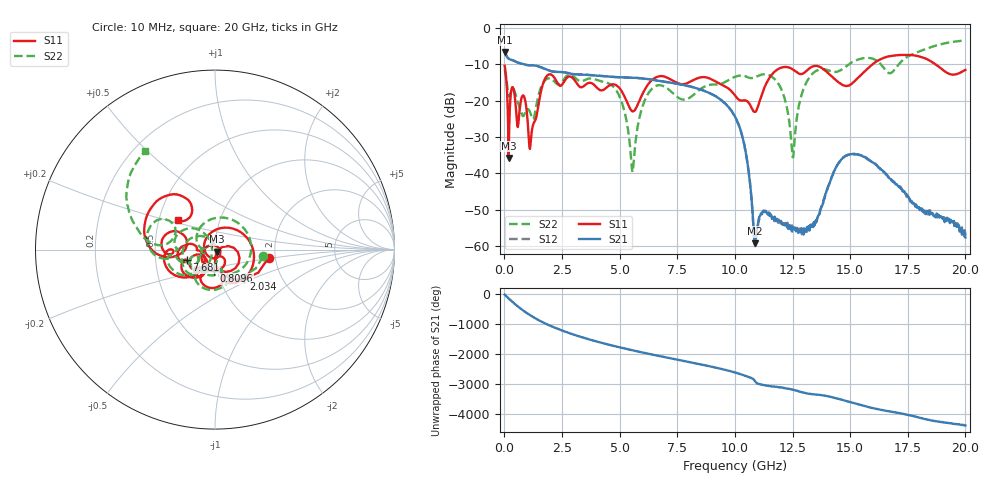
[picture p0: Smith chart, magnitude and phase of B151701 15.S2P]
!  2-Port S-parameters saved by WinCal
! VAR MeasName=S-Parameters (CALIBRATED_DATA) read from VNA (N5244A)
! VAR MeasDate=2015-12-24 19:09:51
! VAR NAME=B151701 15
! VAR FILENAME=B151701 15.S2P
! VAR DATE=2015-12-24 19:09:51
! VAR PHYS_PORTS=1,3
# Hz S DB R 50
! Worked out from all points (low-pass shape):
!   801 points, 10 MHz to 20 GHz, reference 50 ohm
!   highest |S21| = -6.63 dB at 10 MHz (marker M1); lowest = -59.3 dB at 10.85 GHz (marker M2)
!   |S21| within 3 dB of the highest: start of sweep to 635.4 MHz
!   lowest |S11| = -35.7 dB at 184.9 MHz (marker M3), VSWR 1.03, Z = 51.1 - j1.19 ohm
!   |S11| at or under -10 dB: start of sweep to 15.98 GHz; 18.7 GHz to end of sweep
!   |S22| runs from -39.6 to -3.5 dB; largest |S21 - S12| = 0.0013
!   S11 on the Smith chart (normalised r, x): 10 MHz: 1.84, -0.18; 809.6 MHz: 0.96, -0.23; 2.034 GHz: 1.30, -0.44; 7.681 GHz: 0.72, -0.09; 20 GHz: 0.63, +0.22
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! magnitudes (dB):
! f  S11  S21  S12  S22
! 10 MHz  -10.4  -6.6  -6.7  -11.3
! 184.9 MHz  -35.7  -8.4  -8.4  -18.4
! 809.6 MHz  -18.6  -9.9  -9.9  -24.3
! 1.134 GHz  -31.9  -10.3  -10.3  -23.5
! 2.034 GHz  -12.8  -11.9  -11.9  -14.0
! 3.358 GHz  -16.3  -12.8  -12.8  -14.7
! 4.858 GHz  -15.8  -13.5  -13.5  -17.2
! 5.557 GHz  -23.0  -13.7  -13.7  -39.6
! 6.032 GHz  -17.7  -13.9  -13.9  -20.9
! 6.682 GHz  -13.4  -14.5  -14.5  -15.8
! 7.681 GHz  -15.5  -15.6  -15.6  -19.6
! 10.01 GHz  -18.6  -24.4  -24.4  -13.4
! 10.48 GHz  -20.0  -34.6  -34.5  -13.4
! 10.85 GHz  -23.1  -59.3  -59.3  -13.6
! 11.25 GHz  -16.8  -50.4  -50.2  -12.8
! 11.93 GHz  -11.1  -53.2  -53.0  -15.8
! 12.5 GHz  -11.4  -54.8  -55.3  -35.5
! 12.88 GHz  -12.7  -55.1  -55.3  -18.7
! 13.35 GHz  -10.7  -54.2  -54.3  -12.7
! 14.78 GHz  -15.9  -35.3  -35.3  -10.8
! 16.68 GHz  -7.8  -41.2  -41.2  -12.4
! 20 GHz  -11.6  -57.6  -56.9  -3.5
